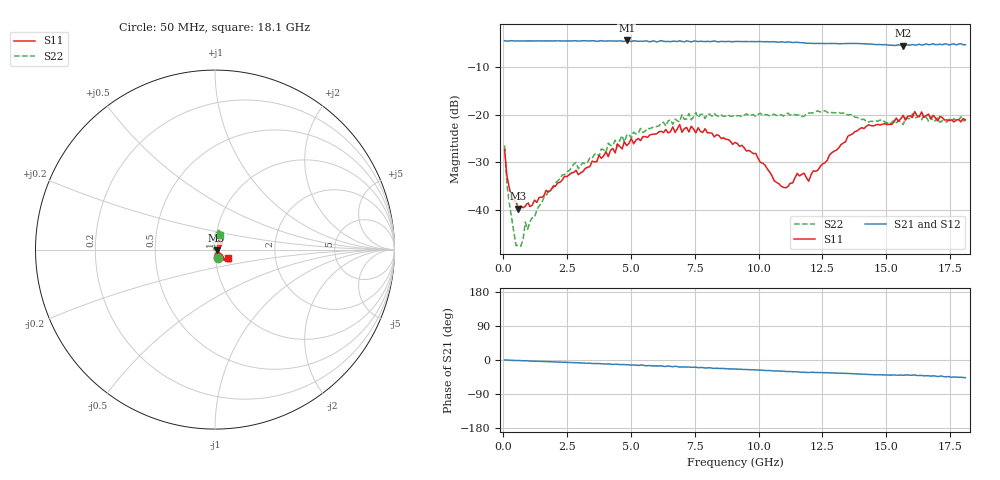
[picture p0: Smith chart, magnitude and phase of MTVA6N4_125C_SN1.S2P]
! Network Analyzer HP8720D.06.14 Serial No. US36140669
!  6 Jul 2005  07:36:49
! Frequency  S11  S21  S12  S22
# HZ  S  DB R 50
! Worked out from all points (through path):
!   201 points, 50 MHz to 18.1 GHz, reference 50 ohm
!   highest |S21| = -4.36 dB at 4.833 GHz (marker M1); lowest = -5.4 dB at 15.66 GHz (marker M2)
!   group delay of S21, straight-line fit = 7.19 ps
!   lowest |S11| = -39.8 dB at 591.5 MHz (marker M3), VSWR 1.02, Z = 50.9 - j0.489 ohm
!   |S11| at or under -10 dB: start of sweep to end of sweep
!   |S22| runs from -47.7 to -19.2 dB; largest |S21 - S12| = 0.018
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5e7  -27.39 -68.7  -4.41 0.1  -4.41 0.2  -26.49 -70.7
1.4025e8  -32.89 -58.3  -4.50 -0.2  -4.47 -0.3  -34.68 -92.5
2.305e8  -35.37 -48.9  -4.45 -0.5  -4.44 -0.5  -38.48 -103.5
5.0125e8  -38.42 -29.8  -4.46 -1.4  -4.44 -1.3  -47.62 -148.3
5.915e8  -39.85 -28.2  -4.43 -1.2  -4.46 -1.3  -47.51 -175.3
7.72e8  -39.62 -15.6  -4.45 -2.1  -4.44 -1.9  -46.40 147.4
8.6225e8  -39.33 -15.2  -4.44 -2.0  -4.46 -2.1  -42.67 152.8
9.525e8  -38.48 -13.3  -4.46 -2.2  -4.44 -2.4  -44.18 132.8
1.76475e9  -36.29 4.9  -4.45 -4.5  -4.43 -4.5  -36.10 99.4
3.1185e9  -32.00 24.5  -4.42 -7.8  -4.47 -8.1  -30.14 98.5
4.83325e9  -26.52 50.2  -4.36 -12.5  -4.43 -13.0  -24.34 80.9
6.09675e9  -23.60 52.9  -4.53 -15.8  -4.43 -15.9  -22.40 79.6
6.909e9  -22.09 59.6  -4.42 -18.7  -4.47 -17.8  -21.52 73.6
9.075e9  -25.84 64.9  -4.57 -23.9  -4.54 -23.9  -20.23 67.5
9.88725e9  -28.16 60.8  -4.62 -26.2  -4.56 -26.3  -20.37 64.2
1.097025e10  -35.31 15.8  -4.68 -29.6  -4.69 -30.0  -20.29 66.0
1.21435e10  -31.84 -37.3  -4.98 -32.5  -4.92 -32.7  -19.60 78.4
1.3768e10  -23.59 -43.6  -4.97 -36.5  -5.01 -36.5  -20.53 80.1
1.512175e10  -22.03 -42.7  -5.38 -39.9  -5.25 -39.9  -22.09 89.0
1.566325e10  -20.15 -36.3  -5.44 -40.3  -5.34 -39.4  -22.12 86.8
1.602425e10  -20.60 -38.7  -5.21 -40.0  -5.34 -41.2  -19.83 80.9
1.81e10  -21.10 -31.4  -5.27 -46.6  -5.38 -46.8  -21.30 71.0
